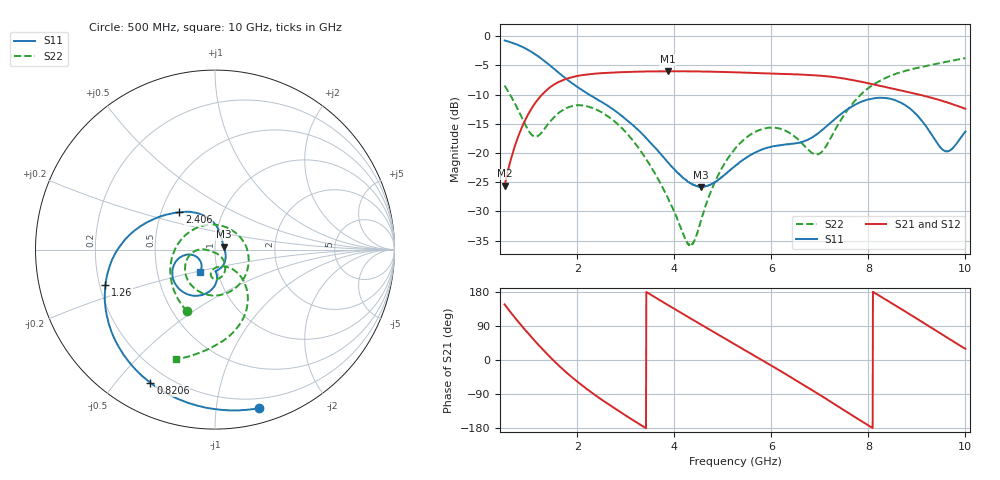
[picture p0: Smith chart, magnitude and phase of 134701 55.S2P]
!  2-Port S-parameters saved by WinCal
! VAR MeasName=S-Parameters (CALIBRATED_DATA) read from VNA (N5242A)
! VAR MeasDate=2013-7-3 16:40:09
! VAR NAME=134701 55
! VAR FILENAME=134701 55.S2P
! VAR DATE=2013-7-3 16:40:09
! VAR PHYS_PORTS=1,2
# Hz S MA R 50
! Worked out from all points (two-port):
!   1601 points, 500 MHz to 10 GHz, reference 50 ohm
!   highest |S21| = -6.01 dB at 3.861 GHz (marker M1); lowest = -25.6 dB at 500 MHz (marker M2)
!   |S21| within 3 dB of the highest: 1.398 GHz to 8.517 GHz (7.119 GHz wide, 144 % of centre)
!   lowest |S11| = -25.8 dB at 4.555 GHz (marker M3), VSWR 1.11, Z = 55.1 + j1.8 ohm
!   |S11| at or under -10 dB: 2.243 GHz to end of sweep
!   |S22| runs from -36.0 to -3.8 dB; largest |S21 - S12| = 0.0029
!   S11 on the Smith chart (normalised r, x): 500 MHz: 0.12, -1.31; 820.6 MHz: 0.13, -0.62; 1.26 GHz: 0.22, -0.15; 2.406 GHz: 0.62, +0.28; 10 GHz: 0.82, -0.21
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5e8  0.9182 -74.6  0.05245 146.8  0.05232 146.7  0.3771 -114.3
8.20625e8  0.825 -115.9  0.1528 94.9  0.1525 94.8  0.2152 175.2
1.064062e9  0.7294 -143.2  0.2434 58.8  0.243 58.7  0.1425 102.8
1.26e9  0.6407 -162.3  0.3118 31.2  0.3116 31.2  0.1487 37.7
1.645938e9  0.4745 168.9  0.4108 -18.1  0.4104 -18.2  0.2252 -43.5
2.085312e9  0.3483 147.2  0.463 -65.8  0.4622 -65.9  0.2555 -98.0
2.405938e9  0.288 133.7  0.4786 -96.2  0.478 -96.2  0.2338 -127.2
3.070938e9  0.1839 103.6  0.4942 -152.6  0.4935 -152.6  0.1393 -169.0
3.670625e9  0.1031 75.6  0.5001 160.2  0.4994 160.2  0.05908 179.3
3.860625e9  0.08358 66.7  0.5005 145.6  0.5002 145.6  0.0418 -175.9
4.305938e9  0.05598 40.0  0.4991 111.8  0.4994 111.9  0.01643 -117.1
4.555312e9  0.05115 18.6  0.498 93.0  0.4985 93.0  0.0268 -62.3
4.87e9  0.05735 -10.8  0.4951 69.4  0.4957 69.5  0.06025 -50.3
5.25e9  0.07707 -40.6  0.4901 41.1  0.4903 41.0  0.1087 -58.1
6.004062e9  0.1134 -79.4  0.4782 -15.2  0.4784 -15.2  0.1651 -87.5
6.835312e9  0.1353 -86.4  0.4642 -79.2  0.4646 -79.1  0.1003 -87.4
7.066875e9  0.1596 -85.9  0.4559 -97.5  0.457 -97.7  0.1055 -62.0
7.6725e9  0.2513 -102.0  0.4209 -146.5  0.4219 -146.7  0.2646 -49.7
8.420625e9  0.2926 -139.2  0.3616 154.4  0.361 154.2  0.4511 -73.9
8.996562e9  0.2123 -165.7  0.3195 109.4  0.3185 109.1  0.5332 -89.6
9.5725e9  0.1041 -150.8  0.275 63.3  0.2739 63.0  0.5988 -101.6
1e10  0.1526 -124.0  0.239 29.4  0.2384 29.1  0.6482 -109.8
